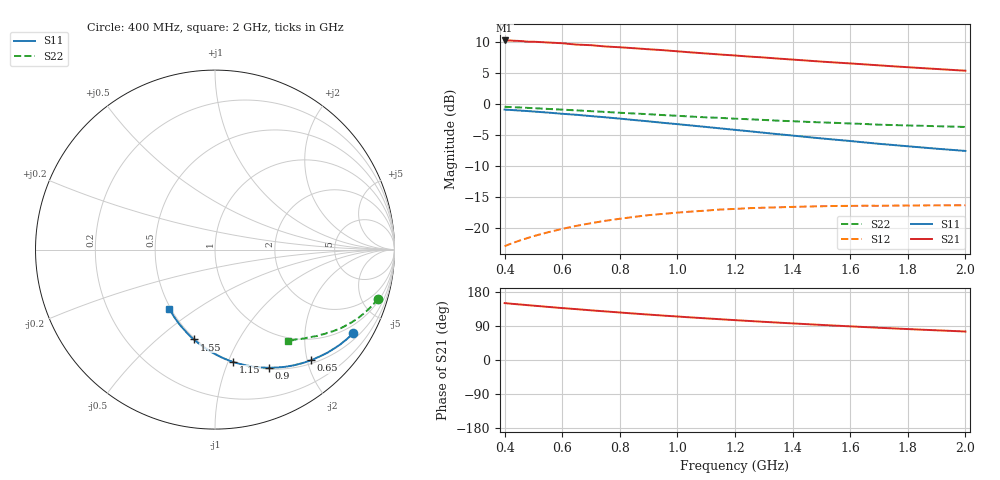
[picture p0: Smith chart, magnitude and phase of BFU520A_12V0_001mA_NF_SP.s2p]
! Filename:  P:\Prog\Test\Noise\ATS_data\Testdata_Net\06 Compressed Noise after Statistics\BFU520A_APG2013_30_A05_12p0V_001mA_NF_CM01_D.sf
! Date/Time: Wed 24/Apr/2013 20:06:20
! BFU520A_APG2013_30_A05_12p0V_1to20mA_NF_CM01_Bias1_R.sf
! Noise Parameter Data File
! BFU520A_APG2013_30_A05_12p0V_1to20mA_NF_CM01
! Date/time: Thu Apr 11 10:46:45 2013
! freq range =  0.4000 to  2.0000 GHz, 37 points
! bias range =  1.0000 to 19.9950 mA, 8 points
! bias supplies used: 1 1 0 0 0 0
! VAR bias_mode= 1  ! Specify V_out, I_out
! VAR bias_var = 1  ! Bias variable = I_out
! VAR V_out= 12.001000
! VAR I_out= 1.000000
! VAR V_in= 0.789700
! VAR I_in= 0.009200
! Device data file deembeded for feedlines and parallel
! Original file: \06 Compressed Noise after Statistics\BFU520A_APG2013_30_A05_12p0V_001mA_NF_CM01_R.sf
! Feed-files: PR017V01_150413_Feed1.s2p, PR017V01_150413_Feed2.s2p
! Parallel-file: PR017V01_150413_Par.s2p
# MHz S MA R 50
!  Freq-MHz  S11-mag  S11-arg  S21-mag  S21-arg  S12-mag  S12-arg  S22-mag  S22-arg
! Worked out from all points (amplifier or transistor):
!   37 points, 400 MHz to 2 GHz, reference 50 ohm
!   highest |S21| = 10.2 dB at 400 MHz (marker M1)
!   |S21| within 3 dB of that: start of sweep to 1.375 GHz
!   unconditionally stable (mu >= 1): nowhere
!   at 500 MHz: K = 0.23, MSG = 15.7 dB, |S12| = -21.3 dB
!   at 1.1 GHz: K = 0.48, MSG = 12.7 dB, |S12| = -17.2 dB
!   at 2 GHz: K = 0.86, MSG = 10.8 dB, |S12| = -16.3 dB
!   lowest NFmin = 0.39 dB at 420 MHz
!   S11 on the Smith chart (normalised r, x): 400 MHz: 0.70, -3.45; 650 MHz: 0.56, -2.07; 900 MHz: 0.52, -1.42; 1.15 GHz: 0.50, -1.04; 1.55 GHz: 0.49, -0.67; 2 GHz: 0.49, -0.39
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400  0.8999 -31.2  3.244 150.1  0.07138 69.8  0.9469 -16.7
440  0.8877 -34.2  3.221 147.4  0.07742 68.1  0.9385 -18.2
460  0.8811 -35.7  3.206 146.1  0.08032 67.3  0.9344 -18.9
480  0.8754 -37.1  3.171 144.7  0.08308 66.3  0.9287 -19.7
500  0.8681 -38.6  3.168 143.4  0.08588 65.6  0.9242 -20.4
550  0.8512 -42.2  3.124 140.2  0.09232 63.5  0.911 -22.1
600  0.8323 -45.8  3.08 137.1  0.09838 61.6  0.8986 -23.7
650  0.8165 -49.1  3.004 134.1  0.1042 59.9  0.8865 -25.2
700  0.7972 -52.6  2.971 131.1  0.1093 58.1  0.8734 -26.7
750  0.7798 -55.8  2.901 128.2  0.1143 56.5  0.8613 -28.2
800  0.7606 -59.2  2.859 125.4  0.1187 55.0  0.8484 -29.5
900  0.723 -65.6  2.755 119.9  0.1269 52.1  0.8259 -32.0
950  0.7038 -68.8  2.709 117.2  0.1299 50.8  0.8124 -33.3
1050  0.669 -74.8  2.596 112.3  0.1357 48.6  0.7895 -35.5
1150  0.6345 -80.8  2.497 107.5  0.1409 46.5  0.771 -37.5
1200  0.6177 -83.7  2.454 105.2  0.1424 45.7  0.7597 -38.6
1350  0.5699 -92.2  2.317 98.6  0.1467 43.6  0.7322 -41.4
1500  0.527 -100.6  2.191 92.6  0.1497 42.0  0.7093 -43.9
1550  0.5143 -103.2  2.153 90.7  0.1505 41.7  0.703 -44.7
1750  0.4662 -114.2  2.007 83.4  0.1515 41.3  0.6753 -47.8
1850  0.4454 -119.4  1.942 80.0  0.1521 41.4  0.6662 -49.2
2000  0.4178 -127.6  1.851 75.2  0.1526 42.3  0.6517 -51.4
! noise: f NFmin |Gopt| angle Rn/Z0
400  0.5088  0.6995  16.49  0.364
460  0.5162  0.6841  20.79  0.3846
600  0.6183  0.6491  26.43  0.3619
800  0.6123  0.615  38.52  0.2909
1000  0.6631  0.6014  47.66  0.276
1200  0.7234  0.5823  57.56  0.2805
1400  0.7661  0.5701  68.5  0.2337
1600  0.7643  0.5551  77.91  0.1926
1800  0.5961  0.5202  93.92  0.1451
2000  0.6951  0.5905  101.7  0.1271
